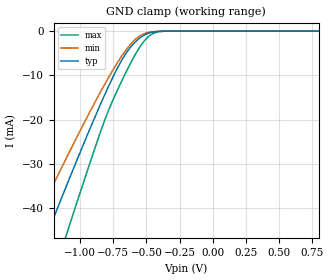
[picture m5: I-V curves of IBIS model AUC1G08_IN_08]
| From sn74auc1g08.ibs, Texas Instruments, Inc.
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[Model]   AUC1G08_IN_08
Model_type  Input
Vinl=0.28
Vinh=0.52
| variable   typ   min   max
C_comp   2.41pF   2.13pF   2.75pF
[Temperature Range]   40   100   -40
| Ambient temperature   25   85   -40
[Voltage range]   0.8   0.8   0.8
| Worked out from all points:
|   GND clamp passes 1 mA (typ) near -0.52 V on its own axis
[GND Clamp]
| AUC1G08_IN_08
|   Voltage   I(typ)   I(min)   I(max)
-3.6V     -228.2mA   -191.9mA   -274.5mA
-1.38V    -55.58mA   -45.51mA   -71.26mA
-1.235V   -44.61mA   -36.51mA   -57.88mA
-1.1V     -34.56mA   -28.31mA   -45.45mA
-1.06V    -31.61mA   -25.93mA   -41.79mA
-830mV    -15.33mA   -12.79mA   -21.29mA
-710mV    -7.815mA   -6.686mA   -12.71mA
-595mV    -2.779mA   -2.171mA   -5.844mA
-535mV    -1.236mA   -834.8uA   -2.942mA
-480mV    -438.2uA   -277.3uA   -1.127mA
-350mV    -14.06uA   -12.12uA   -22.33uA
800mV     155pA      590.8pA    19.39pA
